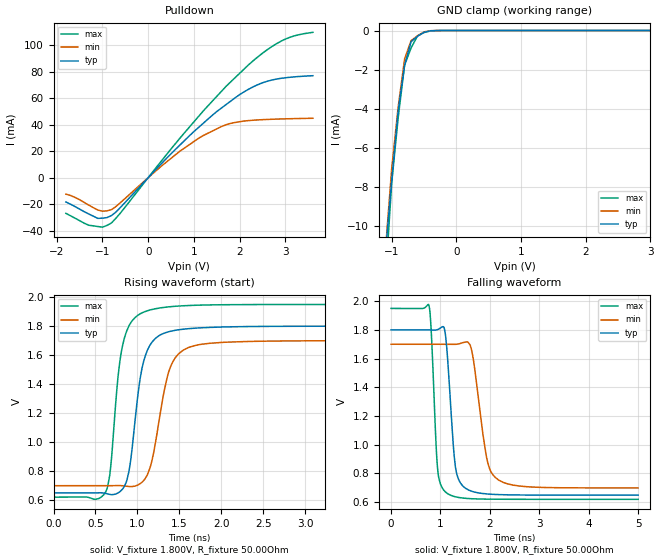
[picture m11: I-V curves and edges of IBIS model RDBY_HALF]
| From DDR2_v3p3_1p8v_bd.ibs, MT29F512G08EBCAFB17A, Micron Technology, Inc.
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| MODEL RDBY_HALF (HALF-Drv RDBY Open-Drain Model)
[Model]   RDBY_HALF
Model_type   Open_drain
Vmeas = 0.900V
Vref = 1.800V
Cref = 50.0pF
Rref = 1000.000Ohm
|   typ   min   max
|C_comp   2.200pF   2.100pF   2.300pF
C_comp_pulldown   2.2000pF   2.1000pF   2.3000pF
[Model Spec]
| Measurement voltage corners
Vmeas   0.900V   0.850V   0.975V
| Timing spec test load voltage corners
Vref   1.800V   1.700V   1.950V
[Voltage Range]   1.8000V   1.7000V   1.9500V
| Junction Temperature (Ambient temp is 35C typ, 70C min, 0C max)
[Temperature Range]   50.0   85.0   0.0
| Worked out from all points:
|   slope of the pulldown table from 0 to 0.27 V, typ, clamps not added: 27.3 ohm
|   GND clamp passes 1 mA (typ) near -0.74 V on its own axis
|   falling waveform, V_fixture 1.800V, R_fixture 50.00Ohm: 20-80 % time 141ps typ, 238ps min, 102ps max; typ from 1.8 V to 0.647 V
|   rising waveform, V_fixture 1.800V, R_fixture 50.00Ohm: 20-80 % time 160ps typ, 199ps min, 140ps max; typ from 0.647 V to 1.8 V
[Pulldown]
|   Voltage   I(typ)   I(min)   I(max)
-1.8V     -18.41mA   -12.49mA   -27mA
-1.3V     -27.47mA   -20.78mA   -35.98mA
-1.1V     -30.81mA   -24.49mA   -36.95mA
-1V       -30.63mA   -25.38mA   -37.43mA
-800mV    -28.6mA    -24.15mA   -34.18mA
700mV     24.84mA    20.14mA    30.07mA
1.2V      40.95mA    31.74mA    50.22mA
1.6V      52.53mA    38.57mA    65.15mA
2.2V      66.9mA     43.11mA    85.44mA
2.7V      73.71mA    44.09mA    98.94mA
3.1V      75.83mA    44.5mA     106mA
3.6V      77.01mA    44.85mA    109.8mA
[GND Clamp]
|   Voltage   I(typ)   I(min)   I(max)
-1.8V     -53.16mA   -50.88mA   -56.12mA
-1.1V     -11.47mA   -11.4mA    -12.96mA
-1V       -7.665mA   -7.052mA   -7.795mA
-900mV    -4.11mA    -3.914mA   -4.46mA
-800mV    -1.758mA   -1.444mA   -1.763mA
-700mV    -571.8uA   -516.6uA   -889.6uA
-600mV    -291.6uA   -266.6uA   -270.3uA
-500mV    -91.41uA   -70uA      -103.5uA
-400mV    -12.02uA   -10.86uA   -23.14uA
-300mV    -2.452uA   -2.465uA   -1.483uA
3.6V      0A         0A         0A
[POWER Clamp]
|   Voltage   I(typ)   I(min)   I(max)
-1.8V     0A         0A         0A
0V        0A         0A         0A
3.6V      0A         0A         0A
[Ramp]
R_load = 50.00Ohm
|   typ   min   max
dV/dt_r   691.800mV/160.118ps 601.837mV/198.570ps 799.324mV/139.955ps
dV/dt_f   691.800mV/140.709ps 601.837mV/238.244ps 799.324mV/101.747ps
[Falling Waveform]
V_fixture = 1.800V
V_fixture_min = 1.700V
V_fixture_max = 1.950V
R_fixture = 50.00Ohm
|   Time   V(typ)   V(min)   V(max)
0s        1.8V       1.7V       1.95V
760ps     1.8V       1.7V       1.977V
810ps     1.8V       1.7V       1.807V
940ps     1.802V     1.7V       836.9mV
1.14ns    1.618V     1.7V       658.6mV
1.3ns     849.9mV    1.7V       635.8mV
1.5ns     696.5mV    1.715V     625.3mV
1.64ns    673.3mV    1.642V     622mV
2.11ns    651.9mV    770.5mV    618.7mV
5ns       647.1mV    697mV      617.9mV
[Rising Waveform]
V_fixture = 1.800V
V_fixture_min = 1.700V
V_fixture_max = 1.950V
R_fixture = 50.00Ohm
|   Time   V(typ)   V(min)   V(max)
0s        647.1mV    697mV      617.9mV
620ps     643.8mV    697.1mV    652.1mV
680ps     635.7mV    697.2mV    818.2mV
820ps     671.6mV    696.7mV    1.656V
900ps     797mV      691.5mV    1.802V
1.06ns    1.522V     723.7mV    1.894V
1.17ns    1.686V     861.6mV    1.915V
1.38ns    1.763V     1.495V     1.934V
1.62ns    1.783V     1.655V     1.943V
5ns       1.8V       1.7V       1.95V
